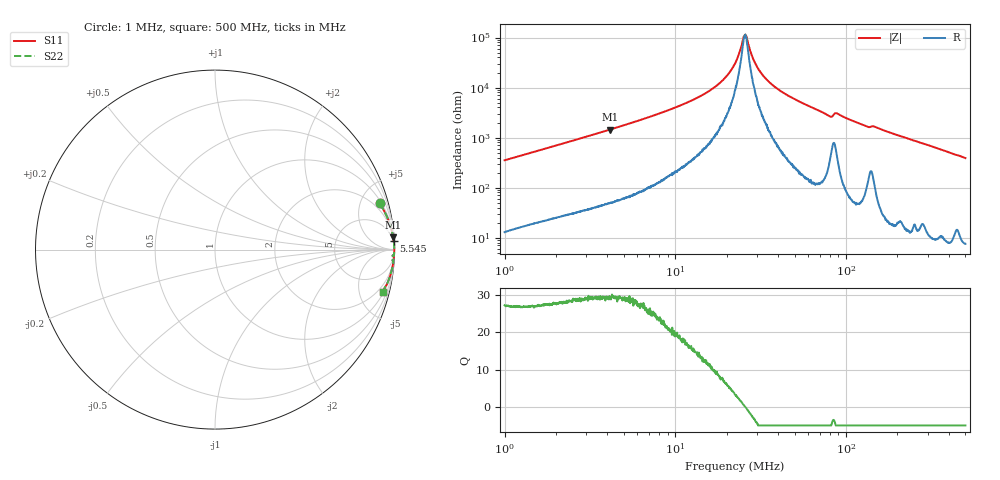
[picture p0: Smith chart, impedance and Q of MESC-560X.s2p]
!s-Parameter Generated by FASTRON Sdn. Bhd.
!FASTRON P/N : MESC-560X
!Keysight Technologies,E4991B,MY54100416,A.01.15
!Date: Fri Mar 27 10:38:10 2026
!Version  : Rev00 Fri Mar 27 10:38:10 2026
!Data & Calibration Information:
!PortZ  Port1:50+j0  Port2:50+j0
!When reading, reference impedance value at option line is always used.
!Remarks : This data is being provided solely for informational purposes.
!Freq	S11	S21	S12	S22
# Hz S dB R 50
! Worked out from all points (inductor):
!   1601 points, 1 MHz to 500 MHz, reference 50 ohm
!   read as one part in series: L = 55.5 uH near 1.032 MHz
!   highest Q = 29.5 at 4.128 MHz (marker M1), where L = 55.6 uH
!   self-resonance near 25.62 MHz
!   S11 on the Smith chart (normalised r, x): 1 MHz: 1.26, +7.04; 5.545 MHz: 2, +39; 500 MHz: 1.15, -7.80
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1000000  -0.42 15.7  -11.36 -72.2  -11.36 -72.2  -0.42 15.7
2820919  -0.08 5.8  -19.89 -82.2  -19.89 -82.2  -0.08 5.8
4127647  -0.04 4.0  -23.23 -84.1  -23.23 -84.1  -0.04 4.0
5545026  -0.03 2.9  -25.94 -85.1  -25.94 -85.1  -0.03 2.9
7957584  -0.02 1.9  -29.54 -85.7  -29.54 -85.7  -0.02 1.9
1.205799e7  -0.01 1.1  -34.39 -85.3  -34.39 -85.3  -0.01 1.1
1.588699e7  -0.01 0.7  -38.78 -84.4  -38.78 -84.4  -0.01 0.7
1.95944e7  -0.01 0.4  -43.99 -80.6  -43.99 -80.6  -0.01 0.4
2.236068e7  -0.01 0.2  -49.72 -72.9  -49.72 -72.9  -0.01 0.2
2.351874e7  -0.01 0.1  -53.23 -65.7  -53.23 -65.7  -0.01 0.1
2.502671e7  -0.01 0.0  -59.67 -30.7  -59.67 -30.7  -0.01 0.0
2.581658e7  -0.01 -0.0  -60.78 11.0  -60.78 11.0  -0.01 -0.0
2.934708e7  -0.01 -0.2  -49.77 74.5  -49.77 74.5  -0.01 -0.2
3.388275e7  -0.01 -0.4  -43.54 82.6  -43.54 82.6  -0.01 -0.4
4.260918e7  -0.01 -0.7  -38.06 86.0  -38.06 86.0  -0.01 -0.7
6.307767e7  -0.01 -1.4  -32.08 86.9  -32.08 86.9  -0.01 -1.4
7.994179e7  -0.04 -2.1  -28.59 81.1  -28.59 81.1  -0.04 -2.1
8.878078e7  -0.04 -1.9  -29.68 80.7  -29.68 80.7  -0.04 -1.9
1.309196e8  -0.04 -3.4  -24.57 83.6  -24.57 83.6  -0.04 -3.4
1.465289e8  -0.05 -3.4  -24.45 82.6  -24.45 82.6  -0.05 -3.4
1.77937e8  -0.04 -4.4  -22.21 84.6  -22.21 84.6  -0.04 -4.4
5e8  -0.32 -14.3  -12.14 74.6  -12.14 74.6  -0.32 -14.3
